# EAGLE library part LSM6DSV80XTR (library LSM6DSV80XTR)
6-axis IMU (inertial measurement unit) with high-g accelerometer, embedded AI, and sensor fusion for wearables and Source: Datasheet
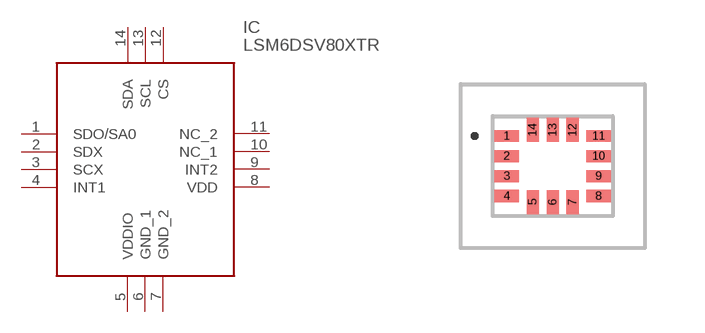
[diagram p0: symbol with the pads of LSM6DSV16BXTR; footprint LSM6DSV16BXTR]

Designator prefix IC

## LSM6DSV80XTR (Arrow_Part_Number: LSM6DSV80XTR; Arrow_Price-Stock: https://www.arrow.com/en/products/lsm6dsv80xtr/stmicroelectronics?utm_currency=USD&region=nac; Description: 6-axis IMU (inertial measurement unit) with high-g accelerometer, embedded AI, and sensor fusion for wearables and; Height: 0.74mm; Manufacturer_Name: STMicroelectronics; Manufacturer_Part_Number: LSM6DSV80XTR)  [LSM6DSV16BXTR]
1  SDO/SA0
2  SDX
3  SCX
4  INT1
5  VDDIO
6  GND_1
7  GND_2
8  VDD
9  INT2
10  NC_1
11  NC_2
12  CS
13  SCL
14  SDA

## Footprint LSM6DSV16BXTR (pad centres in mm)
LGA-14L 2.5 x 3.0 x 0.74 mm XDM)
smd 0.6 x 0.3: 1 -1.15,0.75; 2 -1.15,0.25; 3 -1.15,-0.25; 4 -1.15,-0.75; 8 1.15,-0.75; 9 1.15,-0.25; 10 1.15,0.25; 11 1.15,0.75
smd 0.3 x 0.6: 5 -0.5,-0.9; 6 0,-0.9; 7 0.5,-0.9; 12 0.5,0.9; 13 0,0.9; 14 -0.5,0.9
